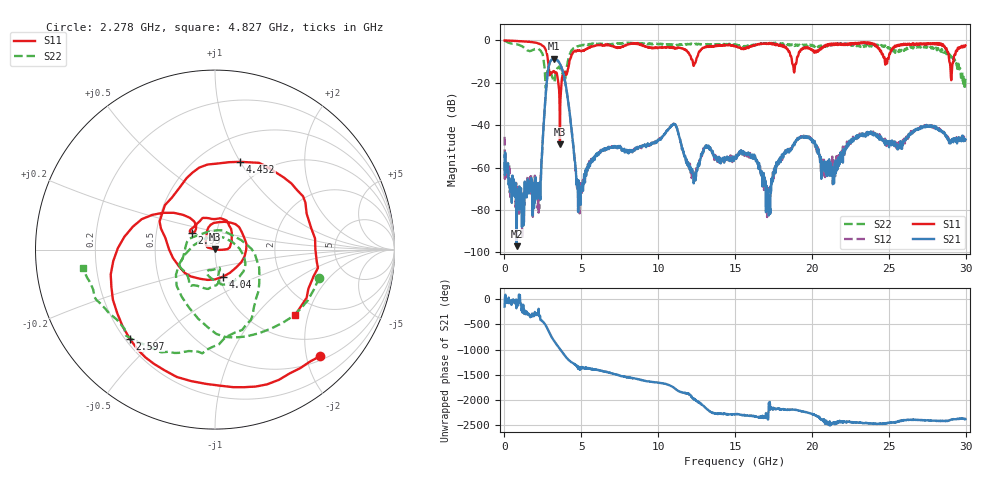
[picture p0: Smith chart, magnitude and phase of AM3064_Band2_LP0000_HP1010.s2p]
# Hz S DB R 50.0
!freq dBS11 angS11 dBS21 angS21 dBS12 angS12 dBS22 angS22
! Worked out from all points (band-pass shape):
!   1600 points, 10 MHz to 29.98 GHz, reference 50 ohm
!   highest |S21| = -8.59 dB at 3.234 GHz (marker M1); lowest = -97.1 dB at 797.2 MHz (marker M2)
!   |S21| within 3 dB of the highest: 2.904 GHz to 3.65 GHz (745.8 MHz wide, 22.8 % of centre)
!   lowest |S11| = -49.1 dB at 3.609 GHz (marker M3), VSWR 1.01, Z = 49.7 + j0.233 ohm
!   |S11| at or under -10 dB: 2.837 GHz to 4.224 GHz (1.387 GHz wide, 39.3 % of centre); 18.7 GHz to 19 GHz (296.8 MHz wide, 1.57 % of centre); 28.94 GHz to 29.2 GHz (258.8 MHz wide, 0.89 % of centre)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
!   |S22| runs from -23.1 to -0.2 dB; largest |S21 - S12| = 0.012
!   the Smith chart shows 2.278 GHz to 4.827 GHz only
!   S11 on the Smith chart (normalised r, x): 2.278 GHz: 0.58, -2.26; 2.597 GHz: 0.22, -0.41; 2.99 GHz: 0.76, +0.14; 4.04 GHz: 1.04, -0.32; 4.452 GHz: 0.76, +1.00; 4.827 GHz: 1.51, -1.66
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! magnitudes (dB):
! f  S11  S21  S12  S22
! 10 MHz  0.0  -54.3  -45.5  -0.2
! 797.2 MHz  -0.3  -97.1  -75.1  -1.9
! 2.278 GHz  -1.6  -67.1  -68.9  -4.4
! 2.597 GHz  -3.3  -34.4  -34.4  -11.7
! 2.99 GHz  -16.0  -9.8  -9.8  -15.1
! 3.234 GHz  -14.6  -8.6  -8.7  -19.6
! 3.609 GHz  -49.1  -11.1  -10.9  -12.9
! 4.04 GHz  -16.1  -23.6  -23.3  -13.0
! 4.452 GHz  -5.9  -47.7  -47.8  -4.1
! 4.827 GHz  -4.8  -66.1  -66.7  -2.6
! 5.015 GHz  -5.1  -68.4  -67.1  -2.4
! 6.383 GHz  -2.4  -51.7  -51.6  -1.8
! 10 GHz  -3.4  -47.2  -46.7  -1.7
! 11.09 GHz  -4.0  -39.6  -39.6  -2.0
! 12.31 GHz  -12.0  -67.4  -63.4  -1.7
! 15 GHz  -2.6  -55.8  -56.0  -1.9
! 16.32 GHz  -2.3  -56.0  -55.2  -2.0
! 17.14 GHz  -1.7  -74.6  -80.6  -1.3
! 19.99 GHz  -4.3  -46.6  -47.1  -2.1
! 21.3 GHz  -2.0  -61.0  -61.3  -1.6
! 25 GHz  -8.3  -48.5  -48.1  -3.2
! 29.98 GHz  -2.4  -46.7  -46.8  -17.3
